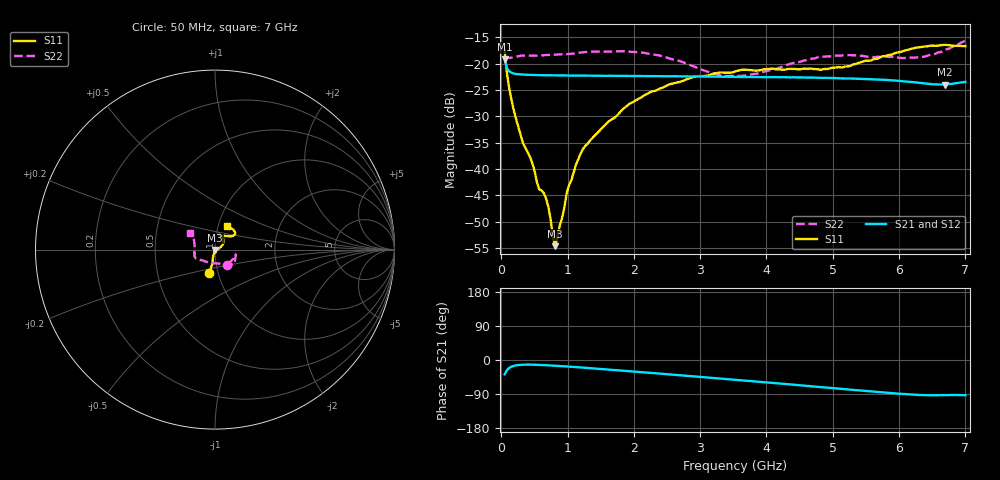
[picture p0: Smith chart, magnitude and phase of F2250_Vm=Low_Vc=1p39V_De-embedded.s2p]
! Integrated Device Technology
! Corporate Headquarters
! 6024 Silver Creek Valley Road
! San Jose, CA 95138  USA
! Phone:  1-408-284-8200
! Toll Free:  1-800-223-1366
! Webpage:  http://www.idt.com/
! Timing and RF Division
! 515 Groton Road, Suite 102
! Westford, MA 01886-6024
! Device:  F2250
! Description: Voltage Variable RF Attenuator
! Frequency:  50.0 -  6000.00 MHz
! Package:  3x3 mm Thin QFN Plastic Package: 16 pin
! Ports:  2 RF, 3 DC
!  Pin  1  = GND
!  Pin  2  = NC
!  Pin  3  = RF1  = Port 1
!  Pin  4  = NC
!  Pin  5  = GND
!  Pin  6  = GND
!  Pin  7  = GND
!  Pin  8  = GND
!  Pin  9  = NC
!  Pin 10  = RF2  = Port 2
!  Pin 11  = NC
!  Pin 12  = GND
!  Pin 13  = GND
!  Pin 14  = VCNTRL
!  Pin 15  = VDD
!  Pin 16  = VMODE
! Vcntrl:  1.390 Volts
! Vmode:  +0.000 Volts
! Vdd:  +3.30  Volts
! Current:  1.193 mA
! Data:  The device was measured on a the F2250 evaluation board which has
!  individual transmission lines to the RF pins.  Data was collected
!  using a calibrated network analyzer.  The evaluation board was
!  de-embedded using a TRL calibration technique.
!  The reference plane is the edge of the package pin.
! Misc:  SN 10
!  Action Tracker AT0258
! Date Measured:  2014-11-26
! Date:  2015-10-15  MJV
! Note:
!  Integrated Device Technology supplies this data as a sample of measured
!  data at the package pin for this product.  Your particular data for this
!  product may vary.
!  Data was taken at 25 degrees C.
!  Integrated Device Technology reserves the right to change this data at anytime.
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# GHz S dB R 50
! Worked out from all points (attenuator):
!   201 points, 50 MHz to 7 GHz, reference 50 ohm
!   highest |S21| = -19.13 dB at 50 MHz (marker M1); lowest = -23.9 dB at 6.687 GHz (marker M2)
!   lowest |S11| = -54.7 dB at 814.5 MHz (marker M3), VSWR 1.00, Z = 50.1 - j0.158 ohm
!   |S11| at or under -10 dB: start of sweep to end of sweep
!   |S22| runs from -22.3 to -15.6 dB; largest |S21 - S12| = 0.00028
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0.05  -17.44 -104.0  -19.13 -38.0  -19.14 -38.1  -19.24 -50.3
0.08475  -21.77 -100.4  -20.85 -26.8  -20.85 -26.8  -18.90 -26.6
0.1195  -24.67 -102.2  -21.43 -20.9  -21.44 -20.9  -18.88 -19.0
0.189  -28.86 -105.1  -21.85 -15.5  -21.84 -15.4  -18.73 -14.5
0.328  -35.11 -106.8  -22.06 -12.4  -22.05 -12.4  -18.44 -13.3
0.467  -38.83 -111.6  -22.12 -12.3  -22.12 -12.3  -18.46 -14.4
0.57125  -43.86 -108.0  -22.16 -12.9  -22.17 -12.9  -18.42 -16.7
0.6755  -45.63 -94.5  -22.18 -13.8  -22.19 -13.8  -18.32 -18.8
0.71025  -47.21 -90.5  -22.18 -14.1  -22.20 -14.1  -18.30 -19.7
0.8145  -54.67 -58.8  -22.20 -15.1  -22.21 -15.1  -18.27 -22.1
0.98825  -44.47 -18.4  -22.23 -17.1  -22.23 -17.1  -18.18 -25.7
1.2315  -36.19 7.9  -22.23 -20.1  -22.23 -20.1  -17.80 -30.2
1.9265  -27.69 28.1  -22.32 -29.5  -22.33 -29.4  -17.68 -38.7
2.37825  -24.78 37.7  -22.37 -35.7  -22.37 -35.7  -18.39 -44.8
2.93425  -22.42 53.3  -22.40 -43.7  -22.41 -43.7  -20.66 -60.0
3.525  -21.47 68.0  -22.50 -52.2  -22.48 -52.2  -22.29 -98.1
4.7065  -20.99 70.1  -22.62 -69.8  -22.64 -69.7  -19.01 -153.2
5.2625  -20.41 51.3  -22.81 -78.2  -22.80 -78.2  -18.35 -162.4
5.85325  -18.31 38.1  -23.12 -86.9  -23.13 -87.0  -18.71 -173.3
6.33975  -16.80 39.3  -23.65 -92.5  -23.66 -92.5  -18.71 168.2
6.68725  -16.40 47.6  -23.94 -92.6  -23.93 -92.7  -17.39 151.9
7  -16.63 62.7  -23.42 -92.9  -23.42 -93.0  -15.56 147.1
